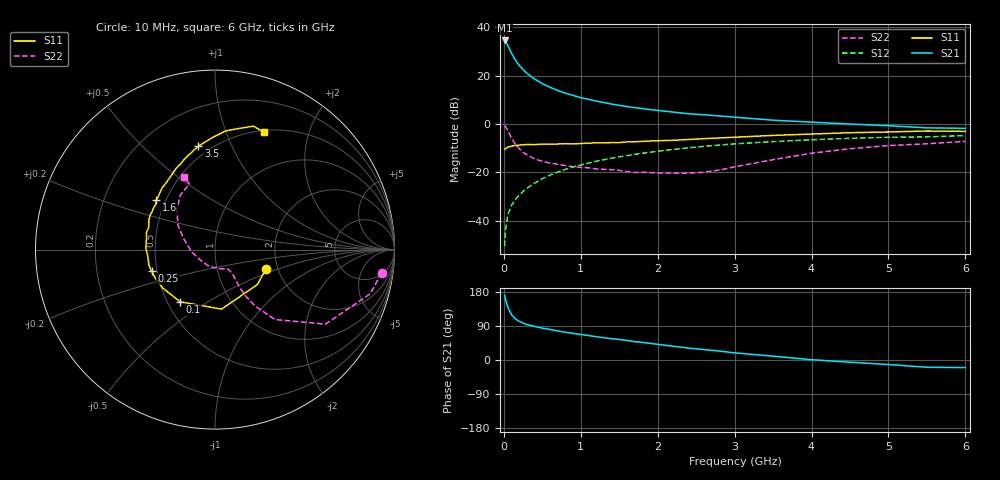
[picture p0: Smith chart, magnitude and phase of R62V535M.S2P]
! SIEMENS Small Signal Semiconductors
! BFR193
! Si NPN RF Bipolar Junction Transistor in SOT23
! VCE = 2.5 V  IC = 35 mA
! Common Emitter S-Parameters:  May  1996
# GHz  S  MA  R  50
!  f  S11  S21  S12  S22
! GHz  MAG  ANG  MAG  ANG  MAG  ANG  MAG  ANG
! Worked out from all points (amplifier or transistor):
!   36 points, 10 MHz to 6 GHz, reference 50 ohm
!   highest |S21| = 34.6 dB at 10 MHz (marker M1)
!   |S21| within 3 dB of that: start of sweep to 65.85 MHz
!   unconditionally stable (mu >= 1): 401.2 MHz to 1.844 GHz
!   at 250 MHz: K = 0.93, MSG = 25.2 dB, |S12| = -27.9 dB
!   at 1.4 GHz: K = 1.02, MAG = 10.3 dB, |S12| = -14.1 dB
!   at 6 GHz: K = 0.95, MSG = 1.5 dB, |S12| = -4.7 dB
!   S11 on the Smith chart (normalised r, x): 10 MHz: 1.73, -0.41; 100 MHz: 0.58, -0.38; 250 MHz: 0.47, -0.13; 1.6 GHz: 0.44, +0.30; 3.5 GHz: 0.43, +0.75; 6 GHz: 0.52, +1.37
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0.01  0.3037 -20.8  53.53 170.5  0.003 80.8  0.9366 -7.9
0.02  0.306 -39.6  51.8 161.5  0.006 78.6  0.9005 -15.8
0.05  0.3338 -83.7  42.85 140.1  0.013 70.0  0.7426 -34.0
0.1  0.3497 -123.8  29.09 119.6  0.021 66.7  0.5133 -49.4
0.15  0.3613 -143.6  21.1 108.4  0.0276 67.7  0.3846 -54.6
0.2  0.3688 -154.1  16.42 101.9  0.0341 69.8  0.3105 -56.5
0.25  0.3729 -161.3  13.33 97.3  0.0404 70.6  0.2603 -56.8
0.3  0.3784 -166.7  11.23 93.8  0.0473 72.0  0.2329 -56.6
0.4  0.3768 -175.6  8.534 88.7  0.0603 72.6  0.1906 -55.2
0.5  0.3851 179.3  6.857 84.1  0.0742 73.0  0.1699 -54.6
0.6  0.3856 174.4  5.767 80.5  0.0884 72.4  0.1561 -54.6
0.7  0.3875 169.7  4.959 76.7  0.1018 71.7  0.1479 -54.9
0.8  0.3942 166.0  4.362 73.2  0.1155 70.6  0.1391 -55.5
1  0.3966 158.0  3.52 67.3  0.143 68.6  0.1275 -58.3
1.1  0.4045 155.5  3.26 64.7  0.1567 67.4  0.125 -61.4
1.4  0.4144 145.6  2.594 56.3  0.1969 63.4  0.1145 -71.5
1.6  0.4285 140.0  2.303 51.5  0.2231 60.5  0.1042 -79.7
2.2  0.4631 125.4  1.773 36.4  0.2995 51.6  0.0971 -115.0
3.5  0.5836 99.2  1.205 10.1  0.4348 31.2  0.1841 160.9
4.5  0.6643 84.8  1.003 -5.8  0.5088 16.9  0.3095 133.0
5.5  0.7205 72.7  0.836 -19.1  0.5445 3.0  0.3926 111.2
6  0.7079 67.2  0.818 -20.0  0.5796 -1.1  0.4391 113.0
